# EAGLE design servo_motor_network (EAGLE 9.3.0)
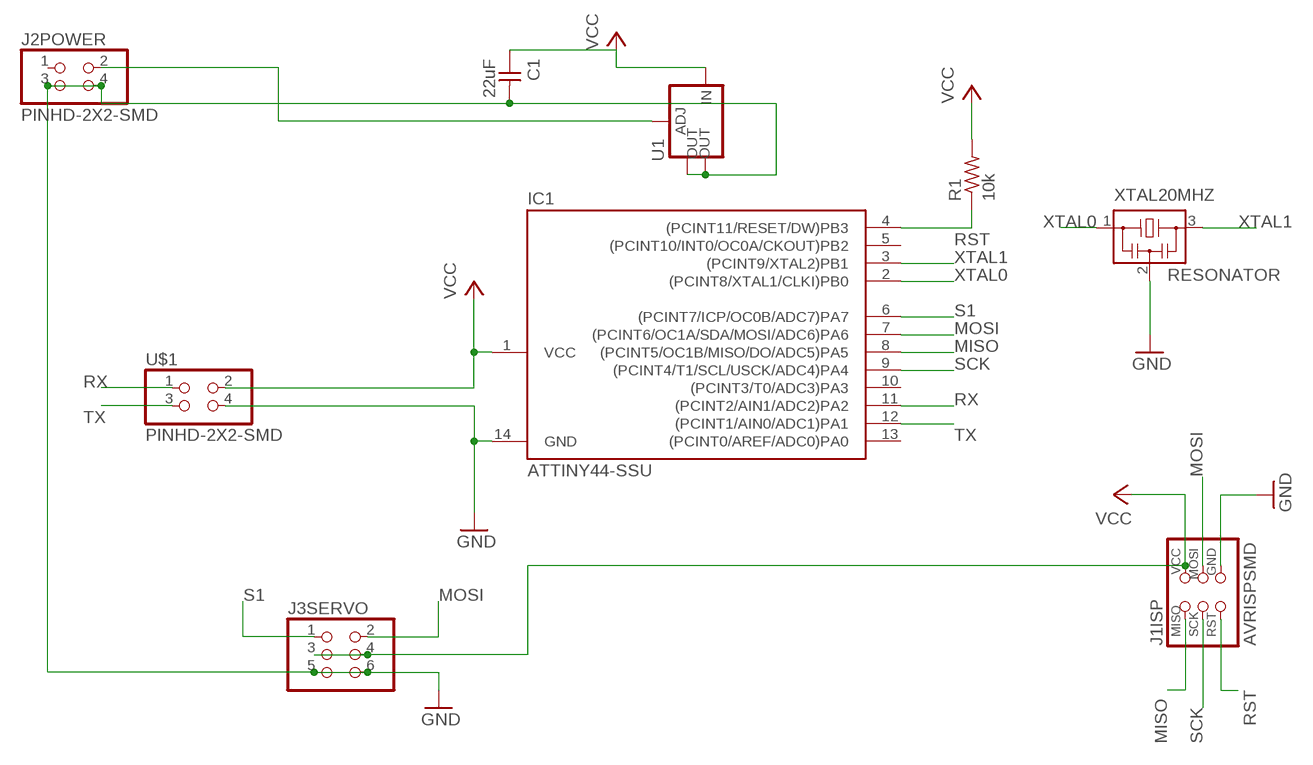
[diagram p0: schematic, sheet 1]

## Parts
C1  22uF  CAP-UNPOLARIZEDFAB  [C1206FAB]
IC1  ATTINY44-SSU  [SOIC14]
J1ISP  AVRISPSMD  [2X03SMD]
J2POWER  PINHD-2X2-SMD  [2X02SMD]
J3SERVO  PINHD-2X3-SMD  [2X03SMD]
R1  10k  RES-US1206FAB  [R1206FAB]
U1  V_REG_LM1117SOT223  [SOT223]
U$1  PINHD-2X2-SMD  [2X02SMD]
XTAL20MHZ  RESONATOR  [EFOBM]

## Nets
GND: C1.2 IC1.14(GND) J1ISP.6(GND) J2POWER.3 J2POWER.4 J3SERVO.5 J3SERVO.6 U1.2(OUT) U1.4(OUT) U$1.4 XTAL20MHZ.2
MISO: IC1.8((PCINT5/OC1B/MISO/DO/ADC5)PA5) J1ISP.1(MISO)
MOSI: IC1.7((PCINT6/OC1A/SDA/MOSI/ADC6)PA6) J1ISP.4(MOSI) J3SERVO.2
N$1: J2POWER.2 U1.1(ADJ)
RST: IC1.4((PCINT11/RESET/DW)PB3) J1ISP.5(RST) R1.1
RX: IC1.11((PCINT2/AIN1/ADC2)PA2) U$1.1
S1: IC1.6((PCINT7/ICP/OC0B/ADC7)PA7) J3SERVO.1
SCK: IC1.9((PCINT4/T1/SCL/USCK/ADC4)PA4) J1ISP.3(SCK)
TX: IC1.12((PCINT1/AIN0/ADC1)PA1) U$1.3
VCC: C1.1 IC1.1(VCC) J1ISP.2(VCC) J3SERVO.3 J3SERVO.4 R1.2 U1.3(IN) U$1.2
XTAL0: IC1.2((PCINT8/XTAL1/CLKI)PB0) XTAL20MHZ.1
XTAL1: IC1.3((PCINT9/XTAL2)PB1) XTAL20MHZ.3
Unconnected: IC1.5((PCINT10/INT0/OC0A/CKOUT)PB2) IC1.10((PCINT3/T0/ADC3)PA3) IC1.13((PCINT0/AREF/ADC0)PA0) J2POWER.1

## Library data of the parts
C1 = fab:CAP-UNPOLARIZED
IC1 = fab:ATTINY44
J1ISP = fab:AVRISP
J2POWER U$1 = fab:PINHD-2X2-SMD
J3SERVO = fab:PINHD-2X3-SMD: PIN HEADER
R1 = fab:RES-US: Resistor (US Symbol)
U1 = fab:V_REG_LM1117: Voltage Regulator LM1117 Standard adjustable voltage regulator but in SMD form. Spark Fun Electronics SKU : COM-00595; PROD_ID: VREG-08170
XTAL20MHZ = fab:RESONATOR

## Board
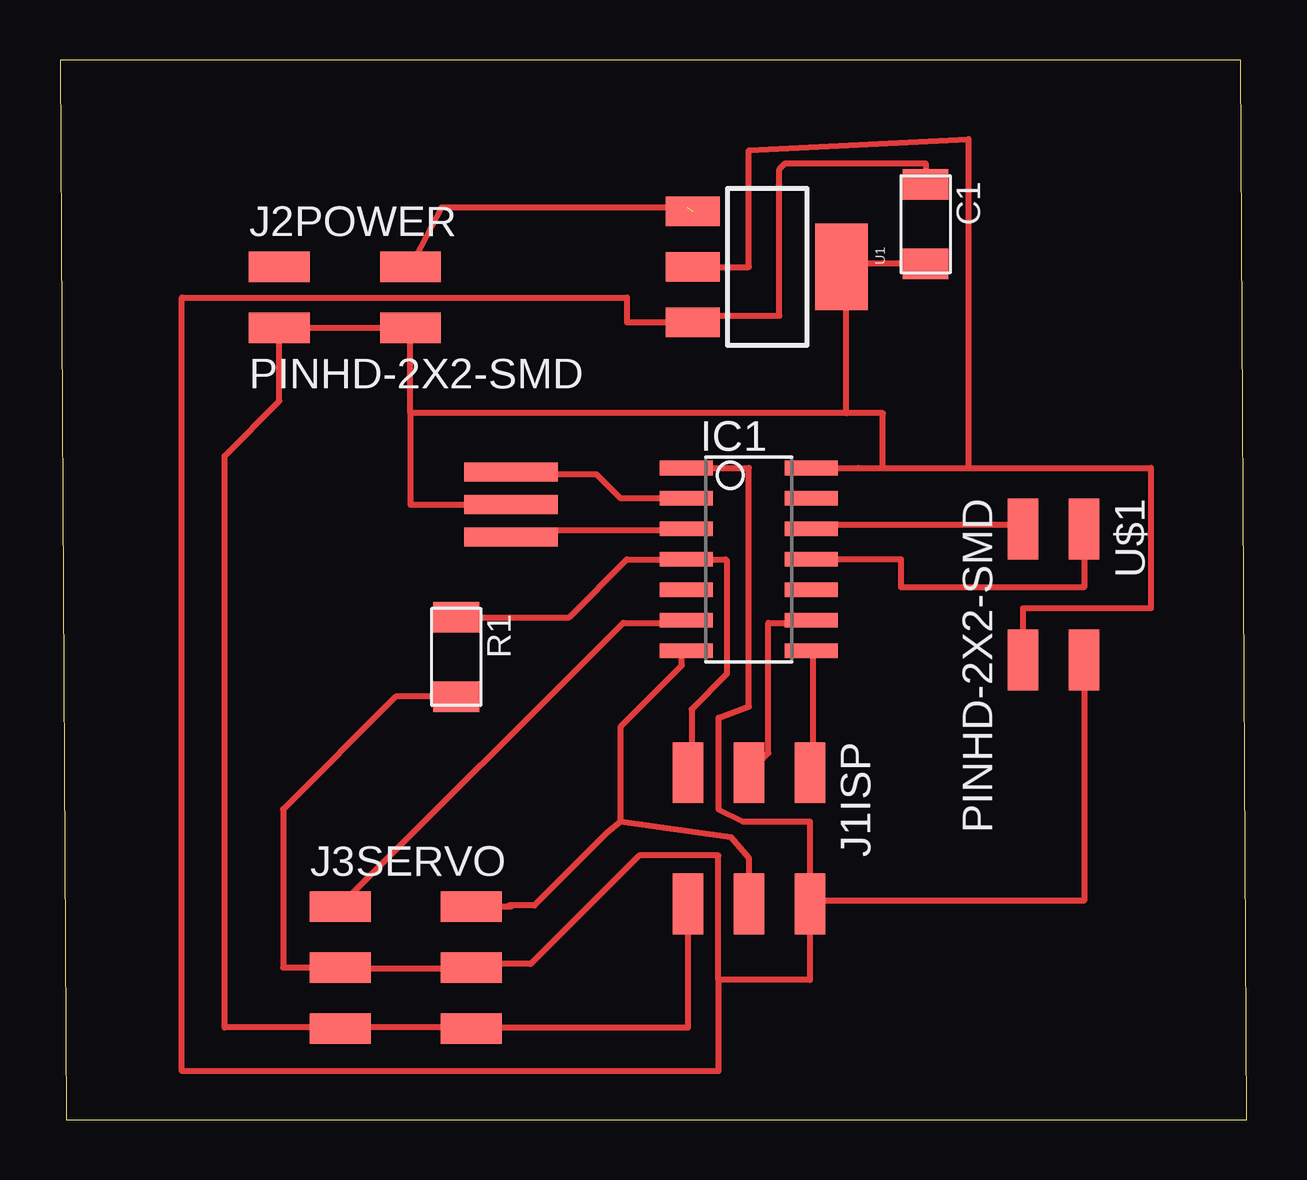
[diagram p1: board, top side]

Size 49.45 x 44.19 mm. Coordinates in mm from the lower left corner, seen from the top.
Outline: 0.25,0 49.45,0 49.2,44.19 0,44.19 0.25,0
Copper layers (1*16): Top 0.035mm / dielectric 1.5mm / Bottom 0.035mm
Design rules "default *": minimum track width 10mil, minimum drill 0.35mm, track to track 6mil, track to pad 6mil, pad to pad 6mil, via to via 6mil, smd to smd 6mil, copper to edge 40mil, drill to drill 6mil, minimum pad ring 10mil, minimum via ring 8mil, stop-mask expansion 4mil, vias tented up to drill 0mil, thermal gap 10mil

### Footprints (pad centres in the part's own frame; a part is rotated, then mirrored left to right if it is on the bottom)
C1206FAB = smd 1.27 x 1.905: 1 -1.651,0; 2 1.651,0
SOIC14 = smd 0.61 x 2.21: 1 -3.81,-2.603; 2 -2.54,-2.603; 3 -1.27,-2.603; 4 0,-2.603; 5 1.27,-2.603; 6 2.54,-2.603; 7 3.81,-2.603; 8 3.81,2.603; 9 2.54,2.603; 10 1.27,2.603; 11 0,2.603; 12 -1.27,2.603; 13 -2.54,2.603; 14 -3.81,2.603
2X03SMD = smd 2.54 x 1.27: 1 -2.54,2.54; 2 2.92,2.54; 3 -2.54,0; 4 2.92,0; 5 -2.54,-2.54; 6 2.92,-2.54
2X02SMD = smd 2.54 x 1.27: 1 -2.54,1.27; 2 2.92,1.27; 3 -2.54,-1.27; 4 2.92,-1.27
R1206FAB = smd 1.27 x 1.905: 1 -1.651,0; 2 1.651,0
SOT223 = smd 1.219 x 2.235: 1 -2.311,-3.099; 2 0,-3.099; 3 2.311,-3.099 | smd 3.6 x 2.2: 4 0,3.099
EFOBM = smd 0.8 x 3.9: 1 -1.35,0; 2 0,0; 3 1.35,0

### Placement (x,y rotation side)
C1  36.07,37.34 270 top
IC1  28.7,23.37 270 top
J1ISP  28.7,11.94 270 top
J2POWER  11.68,34.29 0 top
J3SERVO  14.22,6.35 0 top
R1  16.51,19.3 270 top
U1  29.46,35.56 270 top
U$1  41.4,22.1 270 top
XTAL20MHZ  18.8,25.65 270 top

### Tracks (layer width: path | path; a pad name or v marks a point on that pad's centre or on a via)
GND
  Top 0.254: 31.39,27.23 IC1.14 | U1.4 | 30.58,27.03 31.19,27.03 IC1.14 | 40.13,19.3 U$1.4 40.13,21.34 45.47,21.34 45.47,27.18 37.85,27.18 | 11.68,3.86 16.97,3.86 J3SERVO.6 17.17,3.86 26.16,3.86 J1ISP.6 | 11.68,3.86 6.86,3.86 6.86,27.69 9.14,29.97 J2POWER.3 J2POWER.4 14.6,29.46 | 18.8,25.81 XTAL20MHZ.2 14.6,25.65 14.6,29.46 | 11.68,3.86 J3SERVO.5 | 32.77,29.46 34.29,29.46 34.29,27.18 | 32.77,29.46 32.77,35.56 | 32.77,35.56 U1.4 | 34.29,27.18 33.27,27.18 IC1.14 | U1.2 28.7,35.56 28.7,40.42 37.85,40.89 37.85,27.18 | 34.29,27.18 37.85,27.18 | C1.2 32.89,35.69 32.77,35.56 | 32.77,29.46 14.6,29.46
MISO
  Top 0.254: IC1.8 31.39,19.51 31.39,14.63 J1ISP.1
MOSI
  Top 0.254: 28.55,9.55 28.55,9.14 J1ISP.4 28.7,10.92 27.96,11.79 23.37,12.45 | IC1.7 25.91,19.51 25.91,18.95 23.37,16.41 23.37,12.45 | J3SERVO.2 18.79,8.89 18.69,8.94 19.76,8.94 22.76,11.94 23.37,12.45
N$1  (1 unrouted)
  Top 0.254: 26.13,38.05 15.9,38.05 J2POWER.2
RST
  Top 0.254: J1ISP.5 26.31,14.63 26.31,17.12 27.79,18.59 27.79,23.32 27.74,23.37 IC1.4 23.62,23.37 21.21,20.95 R1.1
RX
  Top 0.254: IC1.11 35.05,23.37 35.05,22.2 42.67,22.2 U$1.1
S1
  Top 0.254: IC1.6 25.91,20.73 23.47,20.73 11.68,8.94 J3SERVO.1
SCK
  Top 0.254: IC1.9 31.19,20.73 29.52,20.73 29.52,15.29 J1ISP.3
TX
  Top 0.254: IC1.12 31.39,24.79 40.13,24.79 U$1.3
VCC
  Top 0.254: 26.11,27.23 IC1.1 28.7,27.18 28.7,17.23 27.43,16.76 27.43,12.95 28.45,12.45 31.24,12.45 J1ISP.2 | 26.11,33.05 U1.3 | U$1.2 42.67,9.14 31.39,9.14 J1ISP.2 | J1ISP.2 31.24,5.84 27.43,5.84 | 27.43,5.84 27.43,11.02 24.13,11.02 19.61,6.5 17.17,6.5 J3SERVO.4 16.97,6.3 11.68,6.3 J3SERVO.3 9.3,6.35 9.3,12.95 14,17.65 R1.2 | U1.3 26.64,33.53 29.97,33.53 29.97,39.62 30.23,39.88 36.07,39.88 C1.1 | 27.43,5.84 27.43,2.03 5.08,2.03 5.08,34.29 23.62,34.29 23.62,33.25 U1.3
XTAL0
  Top 0.254: XTAL20MHZ.1 18.88,26.92 22.35,26.92 23.37,25.91 IC1.2
XTAL1
  Top 0.254: IC1.3 25.91,24.59 19,24.59 18.8,24.38 XTAL20MHZ.3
